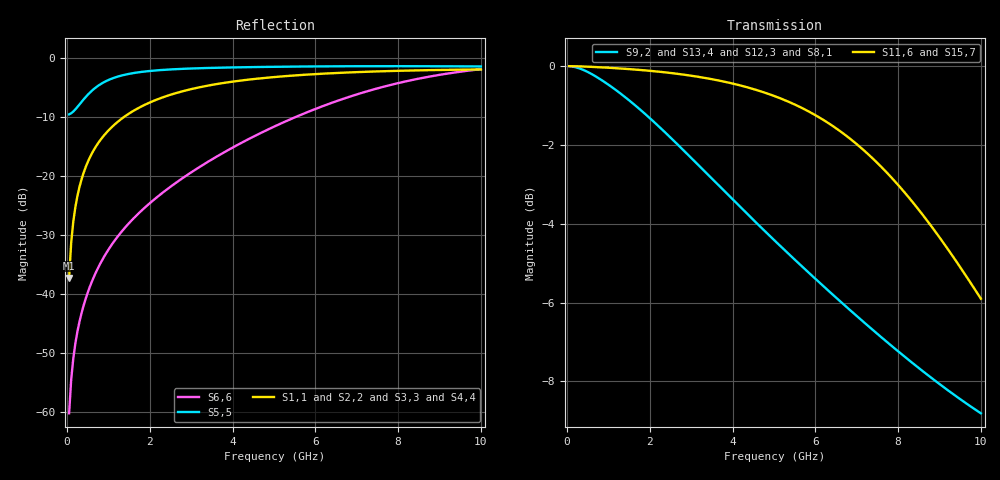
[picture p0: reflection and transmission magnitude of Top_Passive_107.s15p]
! Created Tue Jun  9 07:20:35 2020
! 15 Port Network Data from SP1.SP block
! freq  magS1_1  angS1_1  magS1_2  angS1_2  magS1_3  angS1_3  magS1_4  angS1_4
!  magS1_5  angS1_5  magS1_6  angS1_6  magS1_7  angS1_7  magS1_8  angS1_8
!  magS1_9  angS1_9  magS1_10  angS1_10  magS1_11  angS1_11  magS1_12  angS1_12
!  magS1_13  angS1_13  magS1_14  angS1_14  magS1_15  angS1_15
!  magS2_1  angS2_1
!  magS2_2  angS2_2  magS2_3  angS2_3  magS2_4  angS2_4  magS2_5  angS2_5
!  magS2_6  angS2_6  magS2_7  angS2_7  magS2_8  angS2_8  magS2_9  angS2_9
!  magS2_10  angS2_10  magS2_11  angS2_11  magS2_12  angS2_12  magS2_13  angS2_13
!  magS2_14  angS2_14  magS2_15  angS2_15
!  magS3_1  angS3_1  magS3_2  angS3_2
!  magS3_3  angS3_3  magS3_4  angS3_4  magS3_5  angS3_5  magS3_6  angS3_6
!  magS3_7  angS3_7  magS3_8  angS3_8  magS3_9  angS3_9  magS3_10  angS3_10
!  magS3_11  angS3_11  magS3_12  angS3_12  magS3_13  angS3_13  magS3_14  angS3_14
!  magS3_15  angS3_15
!  magS4_1  angS4_1  magS4_2  angS4_2  magS4_3  angS4_3
!  magS4_4  angS4_4  magS4_5  angS4_5  magS4_6  angS4_6  magS4_7  angS4_7
!  magS4_8  angS4_8  magS4_9  angS4_9  magS4_10  angS4_10  magS4_11  angS4_11
!  magS4_12  angS4_12  magS4_13  angS4_13  magS4_14  angS4_14  magS4_15  angS4_15
!  magS5_1  angS5_1  magS5_2  angS5_2  magS5_3  angS5_3  magS5_4  angS5_4
!  magS5_5  angS5_5  magS5_6  angS5_6  magS5_7  angS5_7  magS5_8  angS5_8
!  magS5_9  angS5_9  magS5_10  angS5_10  magS5_11  angS5_11  magS5_12  angS5_12
!  magS5_13  angS5_13  magS5_14  angS5_14  magS5_15  angS5_15
!  magS6_1  angS6_1
!  magS6_2  angS6_2  magS6_3  angS6_3  magS6_4  angS6_4  magS6_5  angS6_5
!  magS6_6  angS6_6  magS6_7  angS6_7  magS6_8  angS6_8  magS6_9  angS6_9
!  magS6_10  angS6_10  magS6_11  angS6_11  magS6_12  angS6_12  magS6_13  angS6_13
!  magS6_14  angS6_14  magS6_15  angS6_15
!  magS7_1  angS7_1  magS7_2  angS7_2
!  magS7_3  angS7_3  magS7_4  angS7_4  magS7_5  angS7_5  magS7_6  angS7_6
!  magS7_7  angS7_7  magS7_8  angS7_8  magS7_9  angS7_9  magS7_10  angS7_10
!  magS7_11  angS7_11  magS7_12  angS7_12  magS7_13  angS7_13  magS7_14  angS7_14
!  magS7_15  angS7_15
!  magS8_1  angS8_1  magS8_2  angS8_2  magS8_3  angS8_3
!  magS8_4  angS8_4  magS8_5  angS8_5  magS8_6  angS8_6  magS8_7  angS8_7
!  magS8_8  angS8_8  magS8_9  angS8_9  magS8_10  angS8_10  magS8_11  angS8_11
!  magS8_12  angS8_12  magS8_13  angS8_13  magS8_14  angS8_14  magS8_15  angS8_15
!  magS9_1  angS9_1  magS9_2  angS9_2  magS9_3  angS9_3  magS9_4  angS9_4
!  magS9_5  angS9_5  magS9_6  angS9_6  magS9_7  angS9_7  magS9_8  angS9_8
!  magS9_9  angS9_9  magS9_10  angS9_10  magS9_11  angS9_11  magS9_12  angS9_12
!  magS9_13  angS9_13  magS9_14  angS9_14  magS9_15  angS9_15
!  magS10_1  angS10_1
!  magS10_2  angS10_2  magS10_3  angS10_3  magS10_4  angS10_4  magS10_5  angS10_5
!  magS10_6  angS10_6  magS10_7  angS10_7  magS10_8  angS10_8  magS10_9  angS10_9
!  magS10_10  angS10_10  magS10_11  angS10_11  magS10_12  angS10_12  magS10_13  angS10_13
!  magS10_14  angS10_14  magS10_15  angS10_15
!  magS11_1  angS11_1  magS11_2  angS11_2
!  magS11_3  angS11_3  magS11_4  angS11_4  magS11_5  angS11_5  magS11_6  angS11_6
!  magS11_7  angS11_7  magS11_8  angS11_8  magS11_9  angS11_9  magS11_10  angS11_10
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# ghz S ma R 50
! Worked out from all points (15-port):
!   200 points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, 50 MHz to 10 GHz, reference 50 ohm
!   strongest paths, dB at 50 MHz, 2.55 GHz, 5.05 GHz, 7.55 GHz, 10 GHz:
!     S11,6: 0.0, -0.2, -0.8, -2.5, -5.9
!     S15,7: 0.0, -0.2, -0.8, -2.5, -5.9
!     S9,2: 0.0, -1.9, -4.5, -6.8, -8.8
!     S13,4: 0.0, -1.9, -4.5, -6.8, -8.8
!     S12,3: 0.0, -2.0, -4.8, -7.2, -9.2
!     S8,1: 0.0, -2.0, -4.8, -7.2, -9.2
!   lowest |S11| = -37.2 dB at 50 MHz (marker M1), VSWR 1.03, Z = 50 - j1.38 ohm
!   |S11| at or under -10 dB: start of sweep to 1.362 GHz
